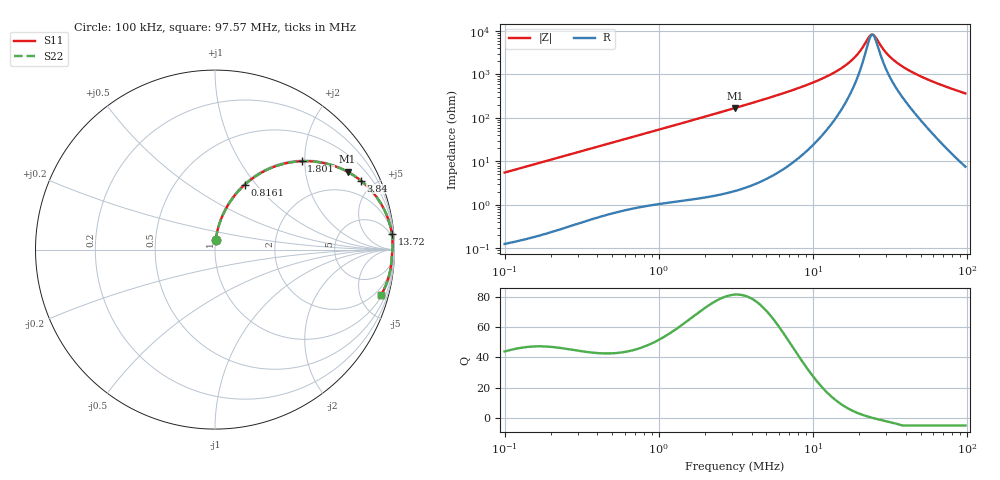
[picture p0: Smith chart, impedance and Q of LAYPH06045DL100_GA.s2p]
! LAYPH06045DL100_GA  S-PARAMETER MODEL  ( General Type )
! Model Generated by TAIYO YUDEN Corporation (http://www.ty-top.com)
! Version 2.0
! TAIYO YUDEN Control No. 180914NI43SB-FBB
! Copyright(c) 2018 TAIYO YUDEN CO.,LTD. All Rights Reserved.
! Product Description (link to TY-COMPAS)
! https://ds.yuden.co.jp/TYCOMPAS/or/detail?pn=LAYPH06045DL100MGA&u=M
! Products Name : Inductors
! Characteristics :
!  Inductance : 10 uH , SRF(min) : -Hz , DC Resistance(max) : 0.0456 Ohm
!  Rated Current : Saturation :2 A , Temp Rise : 1.7 A (25 degC)
!  Case Size : 6.3 x 6.0 / 0.248 x 0.236 [mm/inch] , Thickness : 4.5 / 0.177 [mm/inch]
!  (Conditions: Temperature = 25 degC , DC Bias Current/Voltage = 0A / 0V)
! External Node Assignments :
!  1  o---GGG---o  2
! GND o---------o GND
! Frequency Range : 0.1MHz  -  97.572838MHz  [ 402 STEP ]
# MHz S RI R 50
! Freq[MHz].  S11 Real  S11 Imag  S21 Real  S21 Imag  S12 Real  S12 Imag  S22 Real  S22 Imag
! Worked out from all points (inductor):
!   401 points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, 100 kHz to 97.57 MHz, reference 50 ohm
!   read as one part in series: L = 8.78 uH near 103.5 kHz
!   highest Q = 81.3 at 3.124 MHz (marker M1), where L = 8.62 uH
!   self-resonance near 24.21 MHz
!   S11 on the Smith chart (normalised r, x): 100 kHz: 1.00, +0.11; 816.1 kHz: 1.02, +0.88; 1.801 MHz: 1.03, +1.93; 3.84 MHz: 1.05, +4.20; 13.72 MHz: 3, +22; 97.57 MHz: 1.15, -7.34
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0.1  0.0043 0.055  0.9957 -0.055  0.9957 -0.055  0.0043 0.055
0.316747  0.0327 0.1668  0.9673 -0.1668  0.9673 -0.1668  0.0327 0.1668
0.816104  0.1668 0.3624  0.8332 -0.3624  0.8332 -0.3624  0.1668 0.3624
1.003287  0.2291 0.4107  0.7709 -0.4107  0.7709 -0.4107  0.2291 0.4107
1.801018  0.4826 0.4925  0.5174 -0.4925  0.5174 -0.4925  0.4826 0.4925
3.123665  0.7384 0.4334  0.2616 -0.4334  0.2616 -0.4334  0.7384 0.4334
3.177882  0.7452 0.4297  0.2548 -0.4297  0.2548 -0.4297  0.7452 0.4297
3.840116  0.8119 0.3845  0.1881 -0.3845  0.1881 -0.3845  0.8119 0.3845
5.904422  0.9147 0.2713  0.0853 -0.2713  0.0853 -0.2713  0.9147 0.2713
9.894118  0.9711 0.1506  0.0289 -0.1506  0.0289 -0.1506  0.9711 0.1506
13.72051  0.9849 0.0885  0.0151 -0.0885  0.0151 -0.0885  0.9849 0.0885
18.38301  0.9889 0.0408  0.0111 -0.0408  0.0111 -0.0408  0.9889 0.0408
20.38246  0.989 0.0253  0.011 -0.0253  0.011 -0.0253  0.989 0.0253
22.99163  0.9885 0.00804  0.0115 -0.00804  0.0115 -0.00804  0.9885 0.00804
24.20972  0.9882 0.000822  0.0118 -0.000822  0.0118 -0.000822  0.9882 0.000822
25.49235  0.9878 -0.00632  0.0122 0.00632  0.0122 0.00632  0.9878 -0.00632
28.75564  0.9866 -0.0228  0.0134 0.0228  0.0134 0.0228  0.9866 -0.0228
31.33933  0.9857 -0.0346  0.0143 0.0346  0.0143 0.0346  0.9857 -0.0346
37.87008  0.9834 -0.0615  0.0166 0.0615  0.0166 0.0615  0.9834 -0.0615
48.18621  0.9788 -0.0998  0.0212 0.0998  0.0212 0.0998  0.9788 -0.0998
67.98125  0.9635 -0.1659  0.0365 0.1659  0.0365 0.1659  0.9635 -0.1659
97.57284  0.9264 -0.251  0.0736 0.251  0.0736 0.251  0.9264 -0.251
